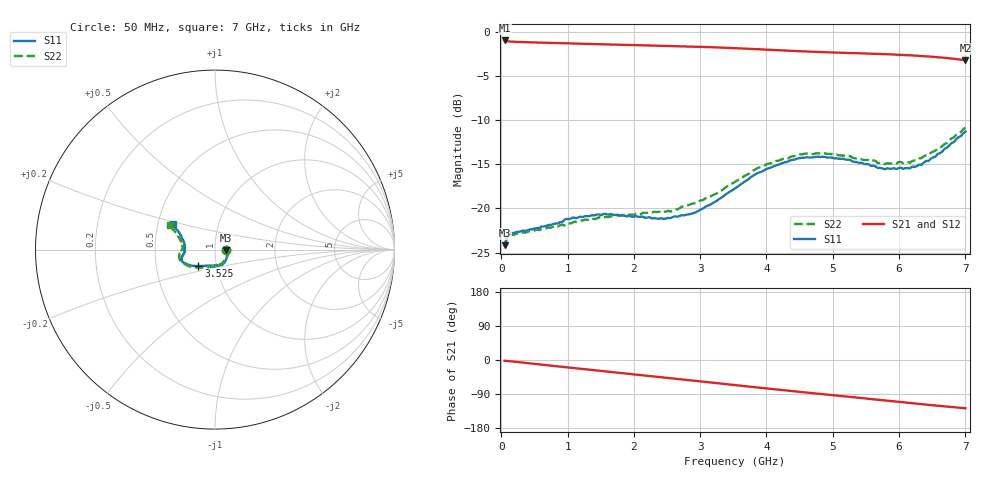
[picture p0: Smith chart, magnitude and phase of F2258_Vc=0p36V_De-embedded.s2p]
! Integrated Device Technology
! Corporate Headquarters
! 6024 Silver Creek Valley Road
! San Jose, CA 95138  USA
! Phone:  1-408-284-8200
! Toll Free:  1-800-223-1366
! Webpage:  http://www.idt.com/
! Timing and RF Division
! 515 Groton Road, Suite 102
! Westford, MA 01886-6024
! Device:  F2258
! Description: Voltage Variable RF Attenuator
! Frequency:  50.0 -  6000.00 MHz
! Package:  3x3 mm Thin QFN Plastic Package: 16 pin
! Ports:  2 RF, 2 DC
!  Pin  1  = NC
!  Pin  2  = NC
!  Pin  3  = RF2  = Port 2
!  Pin  4  = GND
!  Pin  5  = Vdd
!  Pin  6  = NC
!  Pin  7  = VCTRL
!  Pin  8  = NC
!  Pin  9  = GND
!  Pin 10  = RF1  = Port 1
!  Pin 11  = NC
!  Pin 12  = NC
!  Pin 13  = NC
!  Pin 14  = NC
!  Pin 15  = NC
!  Pin 16  = NC
! Vcntrl:  0.360 Volts
! Vdd:  +3.300 Volts
! Current:  1.092 mA
! Data:  The device was measured on a the F2258 evaluation board which has
!  individual transmission lines to the RF pins.  Data was collected
!  using a calibrated network analyzer.  The evaluation board was
!  de-embedded using a TRL calibration technique.
!  The reference plane is the edge of the package pin.
! Misc:  SN 10
!  Action Tracker AT0285
! Date Measured:  2014-12-10
! Date:  2016-01-13  MJV
! Note:
!  Integrated Device Technology supplies this data as a sample of measured
!  data at the package pin for this product.  Your particular data for this
!  product may vary.
!  Data was taken at 25 degrees C.
!  Integrated Device Technology reserves the right to change this data at anytime.
!Freq_(GHz)  S11M_(dB)  S11P_(deg)  S21M_(dB)  S21P_(deg)  S12M_(dB)  S12P_(deg)  S22M_(dB)  S22P_(deg)
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# GHz S dB R 50
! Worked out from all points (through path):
!   201 points, 50 MHz to 7 GHz, reference 50 ohm
!   highest |S21| = -1.00 dB at 50 MHz (marker M1); lowest = -3.2 dB at 7 GHz (marker M2)
!   group delay of S21, straight-line fit = 50.5 ps
!   lowest |S11| = -24.2 dB at 50 MHz (marker M3), VSWR 1.13, Z = 56.6 - j0.404 ohm
!   |S11| at or under -10 dB: start of sweep to end of sweep
!   |S22| runs from -24.3 to -10.8 dB; largest |S21 - S12| = 0.00045
!   S11 on the Smith chart (normalised r, x): 50 MHz: 1.13, -0.01; 3.525 GHz: 0.82, -0.15; 7 GHz: 0.60, +0.18
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0.05  -24.19 -3.3  -1.00 -1.9  -1.00 -1.9  -24.27 -3.1
0.08475  -23.24 -5.6  -1.08 -2.5  -1.08 -2.5  -23.35 -5.3
0.15425  -22.77 -8.7  -1.13 -3.6  -1.13 -3.6  -22.98 -9.2
0.71025  -21.87 -35.4  -1.27 -14.1  -1.27 -14.1  -22.16 -37.5
0.98825  -21.19 -48.8  -1.32 -19.3  -1.32 -19.4  -21.71 -53.2
1.2315  -20.98 -56.9  -1.38 -23.8  -1.38 -23.8  -21.37 -62.2
1.6485  -20.63 -68.4  -1.46 -31.4  -1.46 -31.4  -20.91 -75.3
2.37825  -21.18 -89.2  -1.59 -44.8  -1.59 -44.8  -20.39 -93.1
2.552  -21.10 -95.1  -1.62 -48.0  -1.62 -48.0  -20.36 -98.5
2.93425  -20.44 -111.9  -1.70 -55.1  -1.70 -55.1  -19.42 -111.9
3.247  -19.16 -124.7  -1.78 -61.0  -1.78 -61.0  -18.33 -124.2
3.525  -17.74 -135.4  -1.87 -66.2  -1.87 -66.2  -17.01 -134.8
4.0115  -15.50 -149.6  -2.05 -75.2  -2.05 -75.2  -14.98 -150.3
4.46325  -14.36 -158.2  -2.21 -83.4  -2.21 -83.4  -13.95 -161.5
4.7065  -14.22 -161.5  -2.28 -87.7  -2.28 -87.7  -13.84 -165.8
5.2625  -14.51 -168.4  -2.43 -97.4  -2.43 -97.4  -14.08 -173.9
5.6795  -15.44 -175.1  -2.52 -104.6  -2.52 -104.6  -14.88 -179.4
5.85325  -15.51 -179.2  -2.57 -107.8  -2.57 -107.8  -14.92 176.0
6.166  -15.46 172.9  -2.68 -113.4  -2.68 -113.4  -14.83 170.0
6.33975  -15.05 166.4  -2.76 -116.5  -2.76 -116.5  -14.30 165.6
6.722  -13.14 154.4  -2.99 -123.1  -2.99 -123.1  -12.62 156.5
7  -11.31 148.8  -3.24 -127.4  -3.24 -127.4  -10.85 151.6
